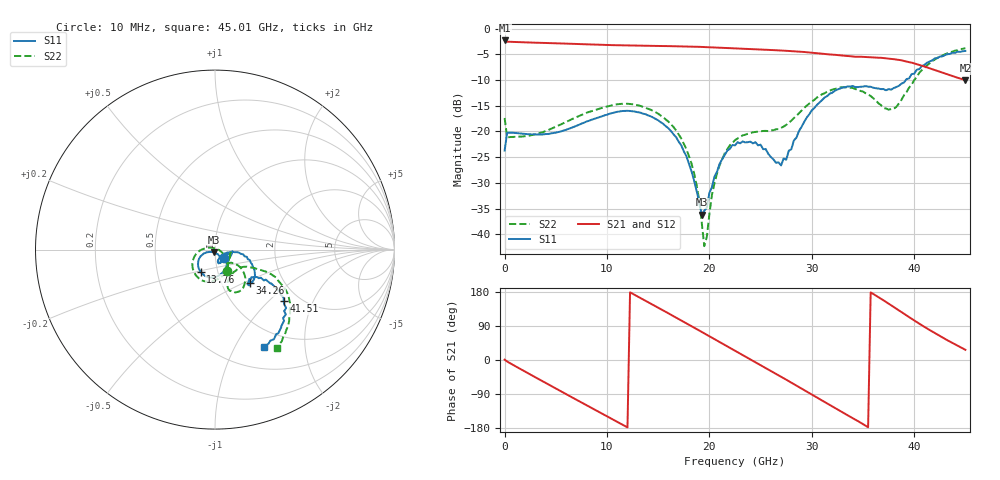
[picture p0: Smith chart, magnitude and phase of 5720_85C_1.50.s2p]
! Device:  ADRF5720
! Description: 0.5dB LSB GaAs MMIC 6-bit Digital Attenuator
! Frequency:  0.000009 -  40 GHz
! Ports:
!	RF1	= Port 1
!	RF2	= Port 2
! Vdd:  3.3 Volt
! Vss:  -3.3 Volt
! Control:  0/3.3 Volt
! State:  1.50 dB attenuation
! Data:  The device was measured using G-S-G Probes on a matrix board.
!  Data was collected using an calibrated 4 port network analyzer.
!  The reference plane for this measurement is at the launchers.
! Note:  Analog Devices supplies this data as a sample of measured data
!  for this product.  Your particular data for this product may vary.
!  Data was taken at 85 degrees C.
!  Analog Devices reserves the right to change this data at anytime.
# GHZ S DB R 45.0
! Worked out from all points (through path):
!   181 points, 10 MHz to 45.01 GHz, reference 45 ohm
!   highest |S21| = -2.30 dB at 10 MHz (marker M1); lowest = -10.0 dB at 45.01 GHz (marker M2)
!   group delay of S21, straight-line fit = 42.7 ps
!   lowest |S11| = -36.2 dB at 19.26 GHz (marker M3), VSWR 1.03, Z = 44.3 - j1.21 ohm
!   |S11| at or under -10 dB: start of sweep to 39.19 GHz
!   |S22| runs from -42.3 to -3.8 dB; largest |S21 - S12| = 0.004
!   S11 on the Smith chart (normalised r, x): 10 MHz: 1.10, -0.10; 13.76 GHz: 0.83, -0.21; 34.26 GHz: 1.36, -0.55; 41.51 GHz: 1.66, -1.24; 45.01 GHz: 0.77, -1.32
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0.01  -23.72 -42.8  -2.30 0.9  -2.29 0.9  -17.37 -60.8
0.26  -20.25 -5.3  -2.54 -4.0  -2.53 -4.0  -21.15 -5.2
4.01  -20.50 -38.9  -2.79 -60.4  -2.77 -60.3  -19.92 -41.1
5.76  -19.82 -49.1  -2.89 -86.3  -2.88 -86.2  -18.38 -55.5
7.76  -18.30 -61.5  -3.03 -115.7  -3.01 -115.6  -16.56 -71.8
10.76  -16.28 -89.7  -3.22 -159.6  -3.20 -159.5  -14.79 -100.9
13.76  -16.63 -123.2  -3.34 156.6  -3.32 156.7  -15.36 -133.3
15.26  -18.21 -140.0  -3.38 134.3  -3.36 134.5  -16.90 -150.9
17.76  -24.79 -160.5  -3.47 96.8  -3.45 97.0  -23.42 177.4
18.76  -31.59 -150.2  -3.52 81.7  -3.51 81.9  -30.39 159.2
19.26  -36.16 -118.7  -3.56 74.1  -3.54 74.3  -37.72 135.3
19.51  -35.42 -100.5  -3.58 70.3  -3.56 70.5  -42.30 95.1
20.76  -27.80 -55.7  -3.68 51.3  -3.66 51.5  -28.12 -19.6
22.76  -22.09 -64.7  -3.87 21.0  -3.85 21.2  -21.38 -44.2
25.01  -22.56 -75.6  -4.07 -13.2  -4.05 -13.0  -19.96 -55.8
27.01  -26.60 -41.2  -4.26 -44.1  -4.24 -43.8  -19.30 -42.7
30.26  -15.42 -13.1  -4.73 -95.2  -4.71 -94.9  -13.85 -38.5
34.26  -11.37 -43.8  -5.47 -157.4  -5.45 -157.1  -11.76 -66.0
37.76  -11.88 -37.1  -5.87 144.3  -5.85 144.7  -15.65 -45.2
39.76  -8.83 -31.4  -6.61 108.9  -6.59 109.3  -10.90 -24.0
41.51  -6.41 -36.9  -7.72 79.2  -7.69 79.6  -6.76 -30.1
45.01  -4.34 -63.2  -10.01 26.9  -9.98 27.2  -3.79 -57.8
